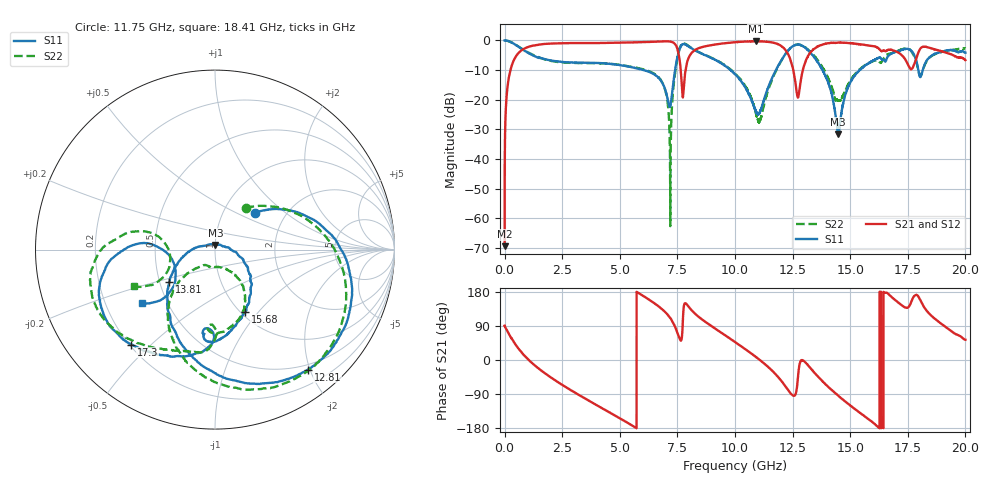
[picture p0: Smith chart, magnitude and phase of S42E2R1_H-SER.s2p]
!{S42E2R1}
!Johanson Technology Inc.
!www.johansontechnology.com
!Test Board Conditions:
!Substrate Type  RO4350B
!Substrate Thickness  50 mil
!Substrate Dk  3.66
!TL Type: GCPW
!TL Trace Width  60 mil
!TL Gap  10 mil
!Electrode orientation  Horizontal
!DUT TOPOLOGY	SERIES
!Mounting Pad LxW  14x55 mil
! Created Wed Nov 25 21:39:03 2020
# khz S ma R 50
! 2 Port Network Data from SP1.SP block
! freq  magS11  angS11  magS21  angS21  magS12  angS12  magS22  angS22
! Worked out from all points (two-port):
!   20001 points, 300 kHz to 20 GHz, reference 50 ohm
!   highest |S21| = -0.29 dB at 10.9 GHz (marker M1); lowest = -69.3 dB at 300 kHz (marker M2)
!   |S21| within 3 dB of the highest: 743 MHz to 7.514 GHz (6.771 GHz wide, 164 % of centre); 8.254 GHz to 12.2 GHz (3.944 GHz wide, 38.6 % of centre)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
!   lowest |S11| = -31.6 dB at 14.48 GHz (marker M3), VSWR 1.05, Z = 50.2 + j2.63 ohm
!   |S11| at or under -10 dB: 6.037 GHz to 7.4 GHz (1.362 GHz wide, 20.3 % of centre); 9.814 GHz to 11.77 GHz (1.958 GHz wide, 18.1 % of centre); 13.8 GHz to 15.41 GHz (1.607 GHz wide, 11 % of centre)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
!   |S22| runs from -62.6 to 0.0 dB; largest |S21 - S12| = 0.02
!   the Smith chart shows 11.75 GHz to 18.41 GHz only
!   S11 on the Smith chart (normalised r, x): 11.75 GHz: 1.40, +0.63; 12.81 GHz: 0.42, -1.97; 13.81 GHz: 0.56, -0.22; 15.68 GHz: 1.05, -0.86; 17.3 GHz: 0.21, -0.43; 18.41 GHz: 0.36, -0.29
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300  0.9995 -0.2  0.0003409 90.3  0.0003974 90.2  1 -0.3
126300  0.9847 -14.2  0.1652 75.5  0.1658 75.5  0.9854 -14.1
453300  0.8569 -47.5  0.5092 42.8  0.5108 42.9  0.8586 -47.3
1482300  0.5087 -113.1  0.8477 -22.7  0.8485 -22.7  0.5228 -112.9
3334300  0.4223 171.3  0.9047 -96.0  0.9038 -96.0  0.4168 176.2
6667300  0.238 66.0  0.9571 142.2  0.956 142.2  0.2427 44.1
7174300  0.07656 110.9  0.9595 112.1  0.9594 112.1  0.01441 8.7
7712300  0.8559 103.2  0.1307 72.5  0.13 72.4  0.8827 95.1
8297300  0.6688 33.7  0.7016 120.5  0.6966 120.5  0.6751 30.1
1.00003e7  0.2707 -39.9  0.9357 47.5  0.9359 47.7  0.2765 -46.2
1.08983e7  0.0648 -24.7  0.9675 8.4  0.9662 8.4  0.06209 -126.3
1.17453e7  0.3003 42.6  0.8993 -36.5  0.8997 -36.4  0.2881 53.7
1.28053e7  0.8452 -52.2  0.1549 -10.5  0.1566 -10.6  0.8436 -60.1
1.33343e7  0.583 -106.0  0.6647 -25.7  0.6642 -26.1  0.6061 -108.8
1.38083e7  0.3116 -144.6  0.858 -56.6  0.8491 -56.7  0.3473 -133.7
1.44833e7  0.02626 84.8  0.9216 -93.9  0.9215 -93.9  0.09693 -97.6
1.56773e7  0.3862 -64.1  0.8351 -150.7  0.8442 -150.7  0.3909 -67.0
1.66673e7  0.5543 -95.1  0.6998 173.7  0.6847 173.5  0.5907 -106.5
1.72963e7  0.7063 -131.5  0.536 141.9  0.5282 142.0  0.7178 -142.7
1.78763e7  0.4489 176.4  0.504 171.9  0.509 172.2  0.4284 166.2
1.84063e7  0.504 -143.6  0.7604 124.0  0.7613 124.6  0.494 -155.9
2e7  0.6206 160.2  0.467 53.3  0.4695 54.3  0.734 135.5
